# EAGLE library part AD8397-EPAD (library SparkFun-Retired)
Rail-to-rail high current output op-amp Retired: IC-10041 Retired: IC-09592
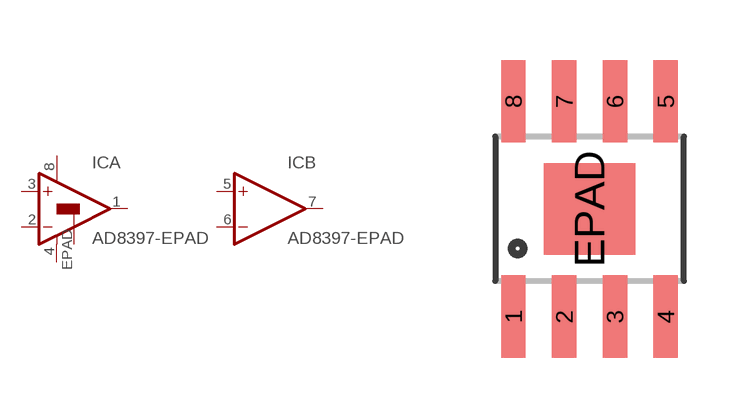
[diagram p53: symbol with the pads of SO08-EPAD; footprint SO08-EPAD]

Designator prefix IC; gates A=OP-AMP+--1 B=OP-AMP-1

## AD8397-EPADEPAD  [SO08-EPAD]
1  A:OUT  out
2  A:-IN  in
3  A:+IN  in
4  A:V-  pwr
5  B:+IN  in
6  B:-IN  in
7  B:OUT  out
8  A:V+  pwr
EPAD  A:EPAD

## Footprint SO08-EPAD (pad centres in mm)
smd 0.61 x 2.057: 1 -1.905,-2.692; 2 -0.635,-2.692; 3 0.635,-2.692; 4 1.905,-2.692; 5 1.905,2.692; 6 0.635,2.692; 7 -0.635,2.692; 8 -1.905,2.692
smd 2.286 x 2.286: EPAD 0,0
